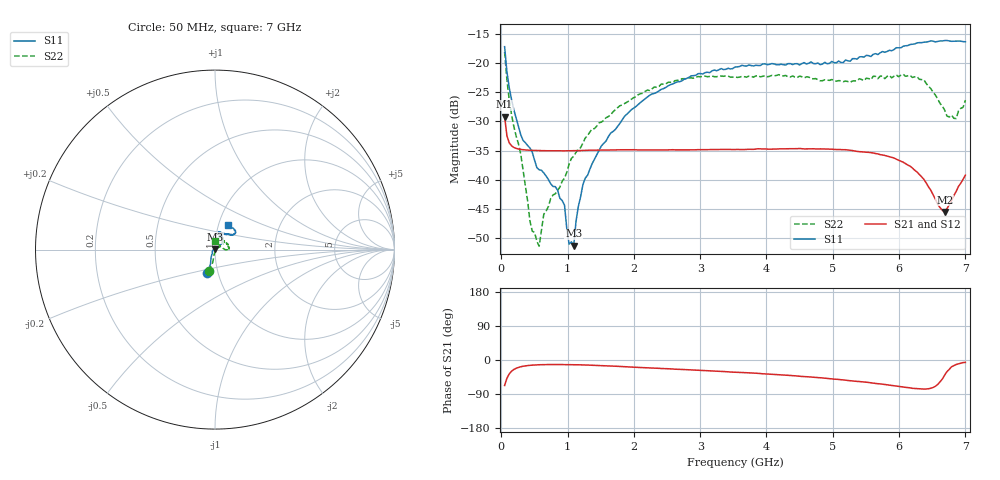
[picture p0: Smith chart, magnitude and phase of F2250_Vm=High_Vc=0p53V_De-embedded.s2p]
! Integrated Device Technology
! Corporate Headquarters
! 6024 Silver Creek Valley Road
! San Jose, CA 95138  USA
! Phone:  1-408-284-8200
! Toll Free:  1-800-223-1366
! Webpage:  http://www.idt.com/
! Timing and RF Division
! 515 Groton Road, Suite 102
! Westford, MA 01886-6024
! Device:  F2250
! Description: Voltage Variable RF Attenuator
! Frequency:  50.0 -  6000.00 MHz
! Package:  3x3 mm Thin QFN Plastic Package: 16 pin
! Ports:  2 RF, 3 DC
!  Pin  1  = GND
!  Pin  2  = NC
!  Pin  3  = RF1  = Port 1
!  Pin  4  = NC
!  Pin  5  = GND
!  Pin  6  = GND
!  Pin  7  = GND
!  Pin  8  = GND
!  Pin  9  = NC
!  Pin 10  = RF2  = Port 2
!  Pin 11  = NC
!  Pin 12  = GND
!  Pin 13  = GND
!  Pin 14  = VCNTRL
!  Pin 15  = VDD
!  Pin 16  = VMODE
! Vcntrl:  0.530 Volts
! Vmode:  +3.300 Volts
! Vdd:  +3.30  Volts
! Current:  1.270 mA
! Data:  The device was measured on a the F2250 evaluation board which has
!  individual transmission lines to the RF pins.  Data was collected
!  using a calibrated network analyzer.  The evaluation board was
!  de-embedded using a TRL calibration technique.
!  The reference plane is the edge of the package pin.
! Misc:  SN 10
!  Action Tracker AT0258
! Date Measured:  2014-11-26
! Date:  2015-10-15  MJV
! Note:
!  Integrated Device Technology supplies this data as a sample of measured
!  data at the package pin for this product.  Your particular data for this
!  product may vary.
!  Data was taken at 25 degrees C.
!  Integrated Device Technology reserves the right to change this data at anytime.
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# GHz S dB R 50
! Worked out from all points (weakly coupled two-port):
!   201 points, 50 MHz to 7 GHz, reference 50 ohm
!   highest |S21| = -29.18 dB at 50 MHz (marker M1); lowest = -45.6 dB at 6.687 GHz (marker M2)
!   lowest |S11| = -51.3 dB at 1.093 GHz (marker M3), VSWR 1.01, Z = 50 + j0.271 ohm
!   |S11| at or under -10 dB: start of sweep to end of sweep
!   |S22| runs from -51.4 to -18.1 dB; largest |S21 - S12| = 6e-05
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0.05  -17.17 -108.4  -29.18 -67.3  -29.18 -67.3  -18.09 -106.8
0.08475  -21.47 -107.3  -32.48 -48.1  -32.48 -48.1  -22.85 -99.6
0.15425  -26.22 -116.5  -34.18 -29.7  -34.19 -29.7  -28.83 -101.2
0.29325  -32.28 -127.2  -34.81 -17.9  -34.81 -17.9  -35.62 -90.8
0.43225  -34.57 -145.1  -34.95 -14.0  -34.95 -14.0  -47.12 -73.6
0.57125  -38.30 -160.9  -35.01 -12.5  -35.01 -12.6  -51.42 -17.7
0.64075  -38.84 -162.2  -35.03 -12.2  -35.02 -12.2  -45.94 16.0
0.9535  -44.38 171.1  -35.05 -12.1  -35.05 -12.1  -39.74 38.7
1.023  -51.07 139.8  -35.04 -12.2  -35.04 -12.2  -37.35 36.0
1.0925  -51.34 87.2  -35.02 -12.4  -35.02 -12.4  -35.97 36.3
1.12725  -47.14 60.1  -35.02 -12.6  -35.02 -12.6  -35.31 32.8
1.2315  -40.83 39.9  -34.98 -13.0  -34.98 -13.0  -33.70 28.5
1.6485  -32.02 41.0  -34.91 -15.9  -34.91 -15.9  -28.89 34.3
1.96125  -27.99 40.7  -34.86 -18.6  -34.86 -18.6  -26.19 34.4
2.37825  -24.75 46.6  -34.89 -22.0  -34.89 -22.0  -23.99 39.8
3.525  -20.66 71.6  -34.83 -32.0  -34.83 -32.1  -22.37 65.0
4.7065  -20.07 71.9  -34.70 -45.6  -34.70 -45.5  -22.69 65.5
5.85325  -17.79 40.5  -36.07 -66.3  -36.07 -66.4  -22.11 15.8
6.3745  -16.40 40.9  -39.96 -76.7  -39.97 -76.9  -22.86 -0.7
6.68725  -16.12 47.8  -45.56 -39.9  -45.53 -39.7  -28.06 21.4
6.861  -16.22 54.5  -42.02 -11.8  -41.99 -11.9  -29.51 59.0
7  -16.33 62.4  -39.23 -6.5  -39.21 -6.7  -26.35 90.3
